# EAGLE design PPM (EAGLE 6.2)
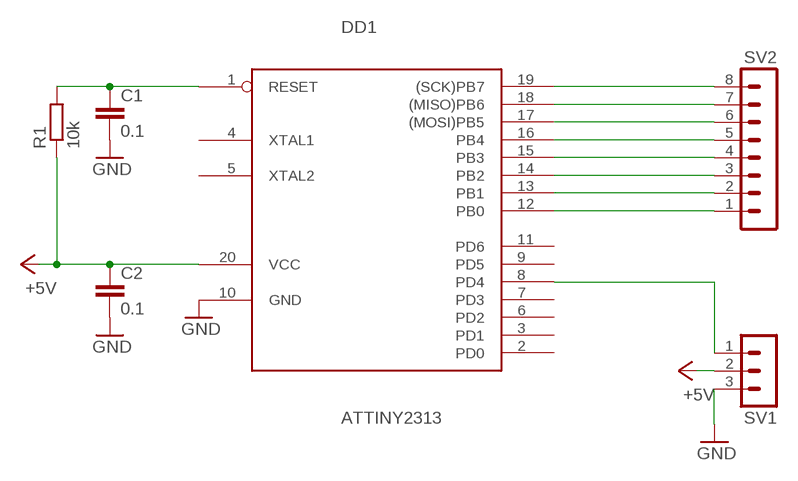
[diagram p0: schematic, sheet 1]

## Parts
C1  0.1  C-EUC1206K  [C1206K]
C2  0.1  C-EUC1206K  [C1206K]
DD1  ATTINY2313  [SO-20LD]
R1  10k  R-EU_R0603  [R0603]
SV1  MA03-1  [MA03-1]
SV2  MA08-1  [MA08-1]

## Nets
+5V: C2.1 DD1.20(VCC) R1.1 SV1.2
GND: C1.2 C2.2 DD1.10(GND) SV1.3
N$1: C1.1 DD1.1(RESET) R1.2
N$2: DD1.12(PB0) SV2.1
N$3: DD1.13(PB1) SV2.2
N$4: DD1.14(PB2) SV2.3
N$5: DD1.15(PB3) SV2.4
N$6: DD1.16(PB4) SV2.5
N$7: DD1.17((MOSI)PB5) SV2.6
N$8: DD1.18((MISO)PB6) SV2.7
N$9: DD1.19((SCK)PB7) SV2.8
N$10: DD1.8(PD4) SV1.1
Unconnected: DD1.2(PD0) DD1.3(PD1) DD1.4(XTAL1) DD1.5(XTAL2) DD1.6(PD2) DD1.7(PD3) DD1.9(PD5) DD1.11(PD6)

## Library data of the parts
C1 C2 = resistor:C-EU: CAPACITOR, European symbol
DD1 = pepelac:ATTINY2313
R1 = resistor:R-EU_: RESISTOR, European symbol
SV1 = con-lstb:MA03-1: PIN HEADER; OC_FARNELL: unknown; OC_NEWARK: unknown
SV2 = con-lstb:MA08-1: PIN HEADER; OC_FARNELL: unknown; OC_NEWARK: unknown

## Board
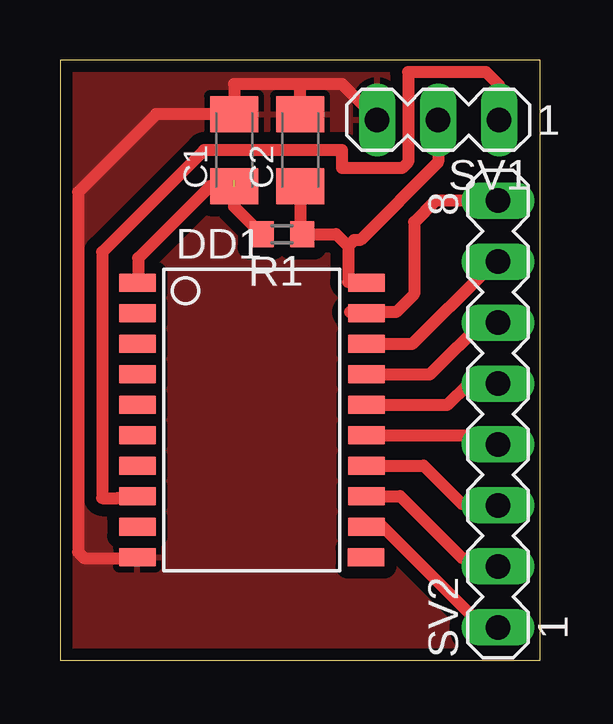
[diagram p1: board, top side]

Size 20 x 25 mm. Coordinates in mm from the lower left corner, seen from the top.
Outline: 0,0 20,0 20,25 0,25 0,0
Copper layers (1*16): Top 0.035mm / dielectric 1.5mm / Bottom 0.035mm
Design rules: minimum track width 6mil, minimum drill 13mil, track to track 6mil, track to pad 6mil, pad to pad 6mil, via to via 6mil, smd to smd 6mil, copper to edge 15mil, drill to drill 8mil, minimum pad ring 10mil, minimum via ring 8mil, stop-mask expansion 4mil, vias tented up to drill 0mil, thermal gap 10mil

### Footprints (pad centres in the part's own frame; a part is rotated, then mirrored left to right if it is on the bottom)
C1206K = smd 1.5 x 2: 1 -1.5,0; 2 1.5,0
SO-20LD = smd 0.762 x 1.524: 1 -5.715,-4.775; 2 -4.445,-4.775; 3 -3.175,-4.775; 4 -1.905,-4.775; 5 -0.635,-4.775; 6 0.635,-4.775; 7 1.905,-4.775; 8 3.175,-4.775; 9 4.445,-4.775; 10 5.715,-4.775; 11 5.715,4.75; 12 4.445,4.775; 13 3.175,4.775; 14 1.905,4.775; 15 0.635,4.775; 16 -0.635,4.775; 17 -1.905,4.775; 18 -3.175,4.775; 19 -4.445,4.775; 20 -5.715,4.775
R0603 = smd 1 x 1.1: 1 -0.85,0; 2 0.85,0
MA03-1 = drill 1.016 long: 1 -2.54,0; 2 0,0; 3 2.54,0
MA08-1 = drill 1.016 long: 1 -8.89,0; 2 -6.35,0; 3 -3.81,0; 4 -1.27,0; 5 1.27,0; 6 3.81,0; 7 6.35,0; 8 8.89,0

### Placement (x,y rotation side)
C1  7.25,21.25 90 top
C2  10,21.25 90 top
DD1  8,10 270 top
R1  9.25,17.74 180 top
SV1  15.75,22.5 180 top
SV2  18.25,10.25 90 top

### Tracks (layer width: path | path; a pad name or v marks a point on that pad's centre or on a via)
+5V
  Top 0.5: 10.25,17.9 R1.1 | R1.1 11.51,17.74 12,17.25 | 12,17.25 12,15.74 DD1.20 | SV1.2 15.75,20.75 12.5,17.5 12.25,17.5 12,17.25 | C2.1 10,17.84 R1.1
GND
  Top 0.5: SV1.3 13.21,22.54 11.75,24 10,24 | C2.2 10,24 | 10,24 7.25,24 C1.2 4,22.75 0.75,19.5 0.75,4.5 1,4.25 3.19,4.25 DD1.10
  pour Top (isolate 0.5): 0,25 20,25 20,0 0,0
N$1  (1 unrouted)
  Top 0.5: 7.88,20.12 7.75,20 7.25,20 | 3,15.74 DD1.1 3.25,15.74 3.25,16.75 6.25,19.75 C1.1 7.25,18.89 R1.2
N$2
  Top 0.5: DD1.12 13.45,5.55 17.25,1.75 17.86,1.75 SV2.1
N$3
  Top 0.5: DD1.13 14.18,6.83 16.75,4.25 17.9,4.25 SV2.2
N$4
  Top 0.5: DD1.14 15.15,8.1 16.75,6.5 18.19,6.5 SV2.3
N$5
  Top 0.5: DD1.15 17.86,9.37 SV2.4
N$6
  Top 0.5: DD1.16 16.14,10.63 17,11.5 18.23,11.5 SV2.5
N$7
  Top 0.5: DD1.17 15.4,11.9 17.75,14.25 18.06,14.25 SV2.6
N$8
  Top 0.5: DD1.18 14.68,13.18 17.75,16.25 17.9,16.25 SV2.7
N$9
  Top 0.5: SV2.8 15.64,19.14 14.75,18.25 14.75,15.25 14,14.5 12.08,14.5 DD1.19
N$10
  Top 0.254: SV1.1 18.29,23.96 | 2.4,6.75 DD1.8
  Top 0.5: 18.29,23.96 17.75,24.5 14.5,24.5 14.5,20.75 14.25,20.5 11.75,20.5 11.75,21.25 6,21.25 1.75,17 1.75,6.75 2.4,6.75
